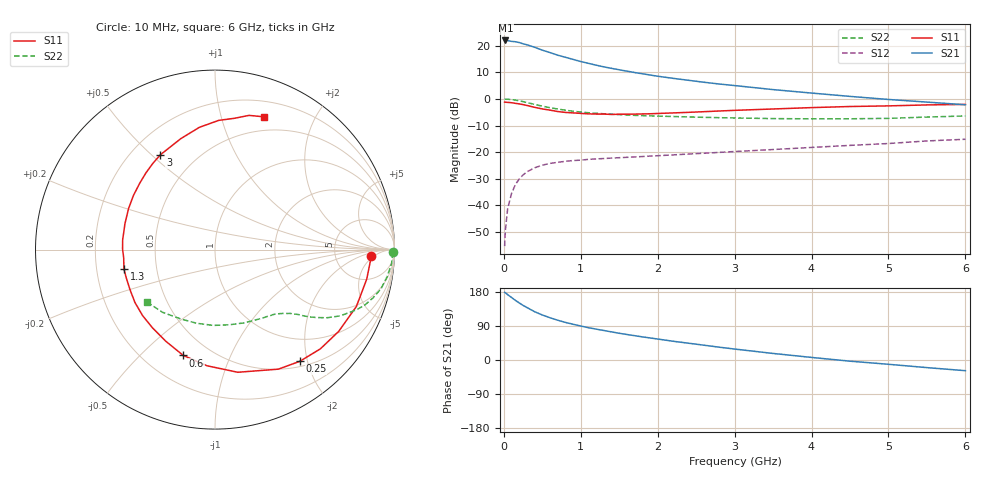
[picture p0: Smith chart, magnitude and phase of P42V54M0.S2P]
! SIEMENS Small Signal Semiconductors
! BFP182
! Si NPN RF Bipolar Junction Transistor in SOT143
! VCE = 2.5 V  IC = 4 mA
! Common Emitter S-Parameters:  March  1996
# GHz  S  MA  R  50
!  f  S11  S21  S12  S22
! GHz  MAG  ANG  MAG  ANG  MAG  ANG  MAG  ANG
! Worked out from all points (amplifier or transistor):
!   36 points, 10 MHz to 6 GHz, reference 50 ohm
!   highest |S21| = 22.0 dB at 20 MHz (marker M1)
!   |S21| within 3 dB of that: start of sweep to 440.4 MHz
!   unconditionally stable (mu >= 1): 1.716 GHz to 5.478 GHz
!   at 250 MHz: K = 0.18, MSG = 24.7 dB, |S12| = -28.6 dB
!   at 1.4 GHz: K = 0.87, MSG = 16.9 dB, |S12| = -22.3 dB
!   at 6 GHz: K = 0.95, MSG = 6.5 dB, |S12| = -15.2 dB
!   S11 on the Smith chart (normalised r, x): 10 MHz: 13, -4; 250 MHz: 0.58, -1.87; 600 MHz: 0.36, -0.68; 1.3 GHz: 0.32, -0.10; 3 GHz: 0.32, +0.53; 6 GHz: 0.35, +1.37
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0.01  0.8706 -2.2  12.38 178.7  0.0017 83.9  0.993 -0.9
0.02  0.8675 -4.5  12.58 177.3  0.0034 89.3  0.9897 -1.8
0.05  0.8613 -11.0  12.54 172.4  0.0087 85.8  0.987 -4.5
0.15  0.8264 -33.4  11.9 157.4  0.0245 72.5  0.9509 -13.2
0.2  0.8065 -43.3  11.49 150.5  0.0312 67.4  0.9214 -16.9
0.25  0.7815 -52.8  10.88 144.1  0.0372 62.8  0.8902 -20.3
0.3  0.7538 -62.1  10.45 138.5  0.0425 58.6  0.8562 -23.1
0.4  0.6951 -79.5  9.371 127.5  0.0506 51.0  0.789 -27.9
0.5  0.6486 -94.0  8.266 118.8  0.0568 45.3  0.7307 -31.3
0.6  0.6155 -106.7  7.445 111.5  0.0613 41.1  0.6845 -33.6
0.7  0.5796 -118.2  6.656 105.0  0.0641 37.9  0.6456 -35.5
0.8  0.5577 -128.8  6.076 99.2  0.0671 35.7  0.614 -36.9
0.9  0.5458 -137.7  5.541 94.3  0.0693 34.0  0.5867 -38.0
1.1  0.5236 -154.6  4.672 85.2  0.073 31.3  0.55 -40.3
1.3  0.519 -167.9  4.011 77.8  0.0757 29.6  0.5254 -42.5
1.6  0.5174 173.8  3.331 67.3  0.0797 28.7  0.4989 -45.9
2.2  0.5454 146.5  2.44 49.5  0.0885 28.4  0.467 -54.2
3  0.6098 119.9  1.784 28.9  0.1025 27.4  0.4386 -68.7
3.5  0.647 107.1  1.498 17.3  0.1117 26.4  0.4263 -79.4
4.5  0.7201 88.4  1.116 -3.1  0.1337 23.0  0.423 -104.0
5.5  0.7713 75.8  0.872 -20.1  0.1621 18.7  0.4558 -130.0
6  0.7884 69.8  0.776 -28.2  0.1743 14.6  0.4787 -142.6
